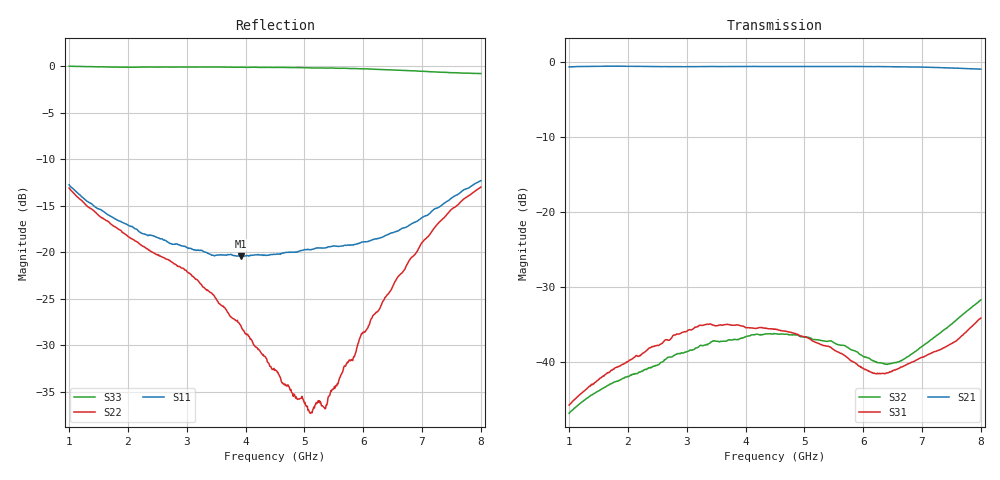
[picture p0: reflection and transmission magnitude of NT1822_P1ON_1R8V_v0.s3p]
! NT1822 PC-P1 ON state
! Port1:PC, Port2:P1, Port3:P2
! VDD=1.8V, VCTL=0V
# hz S ma R 50
! 3 Port Network Data from SP1.SP block
! freq  magS11  angS11  magS12  angS12  magS13  angS13
!  magS21  angS21
!  magS22  angS22  magS23  angS23
!  magS31  angS31  magS32  angS32
!  magS33  angS33
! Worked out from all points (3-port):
!   701 points, 1 GHz to 8 GHz, reference 50 ohm
!   strongest paths, dB at 1 GHz, 2.75 GHz, 4.5 GHz, 6.25 GHz, 8 GHz:
!     S21: -0.6, -0.6, -0.6, -0.6, -0.9
!     S31: -45.8, -36.7, -35.6, -41.6, -34.2
!     S32: -46.9, -39.4, -36.3, -40.2, -31.8
!   lowest |S11| = -20.5 dB at 3.92 GHz (marker M1), VSWR 1.21, Z = 54.9 - j8.71 ohm
!   |S11| at or under -10 dB: start of sweep to end of sweep
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1e9  0.2304 -76.6  0.9311 1.3  0.005133 78.7
     0.9296 1.2  0.2215 -76.6  0.004532 73.7
     0.00513 78.5  0.004518 73.5  1.002 -13.2
2.8e9  0.1105 -70.0  0.9329 -23.9  0.0151 71.0
       0.932 -24.0  0.08621 -91.0  0.01109 69.3
       0.01507 70.8  0.01108 69.3  0.9908 -35.9
3.92e9  0.09486 -56.1  0.9365 -35.6  0.01731 51.1
        0.9352 -35.6  0.04014 -121.4  0.01434 62.1
        0.01735 50.6  0.01431 62.0  0.9893 -49.7
4.5e9  0.09734 -55.5  0.9362 -41.9  0.0165 46.7
       0.9348 -41.9  0.02335 -146.8  0.01538 55.0
       0.01651 46.2  0.01536 54.6  0.9861 -57.7
5.09e9  0.1032 -62.6  0.9371 -48.1  0.01416 40.8
        0.9355 -48.0  0.0137 -150.5  0.01445 49.9
        0.01418 40.4  0.01443 48.9  0.9811 -66.9
5.35e9  0.1054 -68.6  0.9374 -51.1  0.01276 42.9
        0.9363 -50.6  0.01436 -144.5  0.01371 51.1
        0.01279 42.3  0.01369 50.1  0.9784 -71.4
6.17e9  0.1173 -97.9  0.9351 -59.5  0.008451 62.4
        0.9333 -60.1  0.04573 -143.3  0.01016 60.9
        0.008378 61.2  0.01009 60.4  0.9647 -86.9
6.58e9  0.1297 -115.7  0.9326 -64.5  0.008924 84.8
        0.9314 -64.5  0.07297 -147.4  0.009951 82.8
        0.008917 84.2  0.009936 81.7  0.9539 -95.1
7.27e9  0.1735 -146.2  0.9211 -72.4  0.01188 106.7
        0.9195 -72.7  0.1426 -151.8  0.01513 106.8
        0.01187 106.3  0.01516 106.6  0.9314 -108.2
8e9  0.2425 -170.3  0.8989 -80.8  0.01958 125.4
     0.8974 -80.8  0.2241 -152.9  0.02582 113.7
     0.01956 124.8  0.02585 113.0  0.914 -119.5
